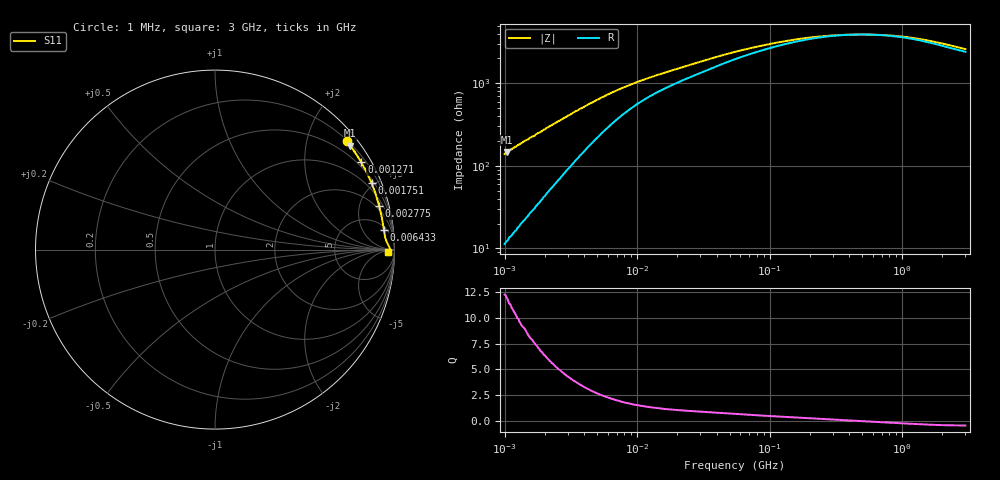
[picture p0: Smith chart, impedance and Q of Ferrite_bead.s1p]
#  HZ  Z  MA  R  50.0
! Measurement of a SMT chip ferrite bead with 60 ohms @ 100 MHz
! (Murata BLM21PG600SN1D)
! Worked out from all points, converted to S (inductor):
!   401 points, 1 MHz to 3 GHz, reference 50 ohm
!   read as one part to ground: L = 22.3 uH near 1.041 MHz
!   highest Q = 11.9 at 1.041 MHz (marker M1), where L = 22.4 uH
!   self-resonance near 516.5 MHz
!   S11 on the Smith chart (normalised r, x): 1 MHz: 0.23, +2.78; 1.271 MHz: 0.36, +3.60; 1.751 MHz: 0.66, +4.84; 2.775 MHz: 1.58, +7.35; 6.433 MHz: 6, +14; 3 GHz: 48, -19
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1000000  2.786 85.3
1020218  2.89 85.3
1040844  2.938 85.2
1061887  2.96 85.1
1127605  3.154 84.8
1173660  3.312 84.6
1271492  3.616 84.2
1377479  3.896 83.7
1433740  4.051 83.5
1751453  4.885 82.2
2139570  5.91 80.5
2412589  6.599 79.3
2775447  7.519 77.9
3323290  8.911 75.7
4225536  10.96 72.3
5161903  12.93 69.1
6433254  15.41 65.3
7400828  17.01 62.7
9410094  19.91 58.4
1.172775e7  22.69 54.7
1.461624e7  25.51 51.3
2.013356e7  29.98 47.3
3.254976e7  37.94 42.0
5.587962e7  48.43 35.1
1.520175e8  67.35 20.6
4.135554e8  77.73 3.8
1.10276e9  72.29 -12.6
3e9  51.83 -21.9
